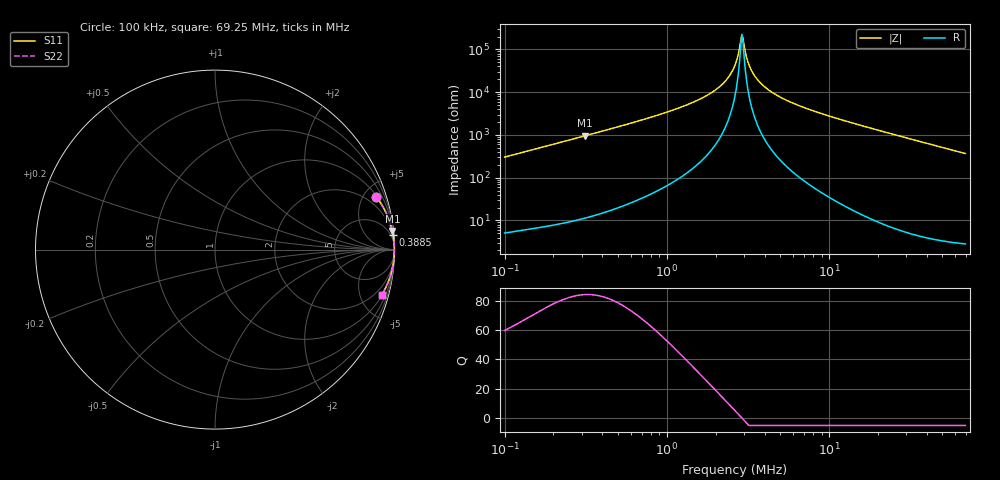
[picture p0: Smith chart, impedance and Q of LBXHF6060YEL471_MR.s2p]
! LBXHF6060YEL471_MR  S-PARAMETER MODEL  ( General Type )
! Model Generated by TAIYO YUDEN Corporation (http://www.ty-top.com)
! Version 1.0
! TAIYO YUDEN Control No. 200120NI43SB-FBB
! Copyright(c) 2020 TAIYO YUDEN CO.,LTD. All Rights Reserved.
! Product Description (link to TY-COMPAS)
! https://ds.yuden.co.jp/TYCOMPAS/or/detail?pn=LBXHF6060YEL471MMR&u=M
! Products Name : Inductors
! Characteristics :
!  Inductance : 470 uH , SRF(min) : 2.0 MHz , DC Resistance(max) : 2.76 Ohm
!  Rated Current : Saturation :450 mA , Temp Rise : 220 mA
!  Case Size : 6.0 x 6.0 / 0.236 x 0.236 [mm/inch] , Thickness : 4.5 / 0.177 [mm/inch]
!  (Conditions: Temperature = 25 degC , DC Bias Current/Voltage = 0A / 0V)
! External Node Assignments :
!  1  o---GGG---o  2
! GND o---------o GND
! Frequency Range : 0.1MHz  -  69.245953MHz  [ 402 STEP ]
# MHz S RI R 50
! Freq[MHz].  S11 Real  S11 Imag  S21 Real  S21 Imag  S12 Real  S12 Imag  S22 Real  S22 Imag
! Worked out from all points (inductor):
!   401 points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, 100 kHz to 69.25 MHz, reference 50 ohm
!   read as one part in series: L = 481 uH near 103.3 kHz
!   highest Q = 84.1 at 314.1 kHz (marker M1), where L = 485 uH
!   self-resonance near 2.903 MHz
!   S11 on the Smith chart (normalised r, x): 100 kHz: 1.10, +6.06; 388.5 kHz: 1, +24; 69.25 MHz: 1.06, -7.33
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0.1  0.8979 0.2945  0.1021 -0.2945  0.1021 -0.2945  0.8979 0.2945
0.299065  0.9868 0.1083  0.0132 -0.1083  0.0132 -0.1083  0.9868 0.1083
0.314101  0.988 0.1031  0.012 -0.1031  0.012 -0.1031  0.988 0.1031
0.388492  0.992 0.0833  0.008 -0.0833  0.008 -0.0833  0.992 0.0833
0.894401  0.9983 0.0336  0.00172 -0.0336  0.00172 -0.0336  0.9983 0.0336
1.390781  0.9992 0.0185  0.000842 -0.0185  0.000842 -0.0185  0.9992 0.0185
1.897481  0.9994 0.0101  0.00057 -0.0101  0.00057 -0.0101  0.9994 0.0101
2.308816  0.9995 0.00533  0.000484 -0.00533  0.000484 -0.00533  0.9995 0.00533
2.505499  0.9995 0.00342  0.000464 -0.00342  0.000464 -0.00342  0.9995 0.00342
2.631463  0.9995 0.00229  0.000455 -0.00229  0.000455 -0.00229  0.9995 0.00229
2.718937  0.9995 0.00154  0.000451 -0.00154  0.000451 -0.00154  0.9995 0.00154
2.855631  0.9996 0.000414  0.000447 -0.000414  0.000447 -0.000414  0.9996 0.000414
2.902706  0.9996 3.9e-05  0.000446 -3.9e-05  0.000446 -3.9e-05  0.9996 3.9e-05
2.999198  0.9996 -0.000711  0.000446 0.000711  0.000446 0.000711  0.9996 -0.000711
3.149982  0.9996 -0.00184  0.000447 0.00184  0.000447 0.00184  0.9996 -0.00184
3.308347  0.9995 -0.00297  0.000451 0.00297  0.000451 0.00297  0.9995 -0.00297
3.531953  0.9995 -0.00449  0.000461 0.00449  0.000461 0.00449  0.9995 -0.00449
3.832833  0.9995 -0.00641  0.000481 0.00641  0.000481 0.00641  0.9995 -0.00641
5.061004  0.9994 -0.0134  0.000617 0.0134  0.000617 0.0134  0.9994 -0.0134
7.869792  0.9988 -0.0268  0.00116 0.0268  0.00116 0.0268  0.9988 -0.0268
23.53582  0.9911 -0.0906  0.00888 0.0906  0.00888 0.0906  0.9911 -0.0906
69.24595  0.929 -0.253  0.071 0.253  0.071 0.253  0.929 -0.253
